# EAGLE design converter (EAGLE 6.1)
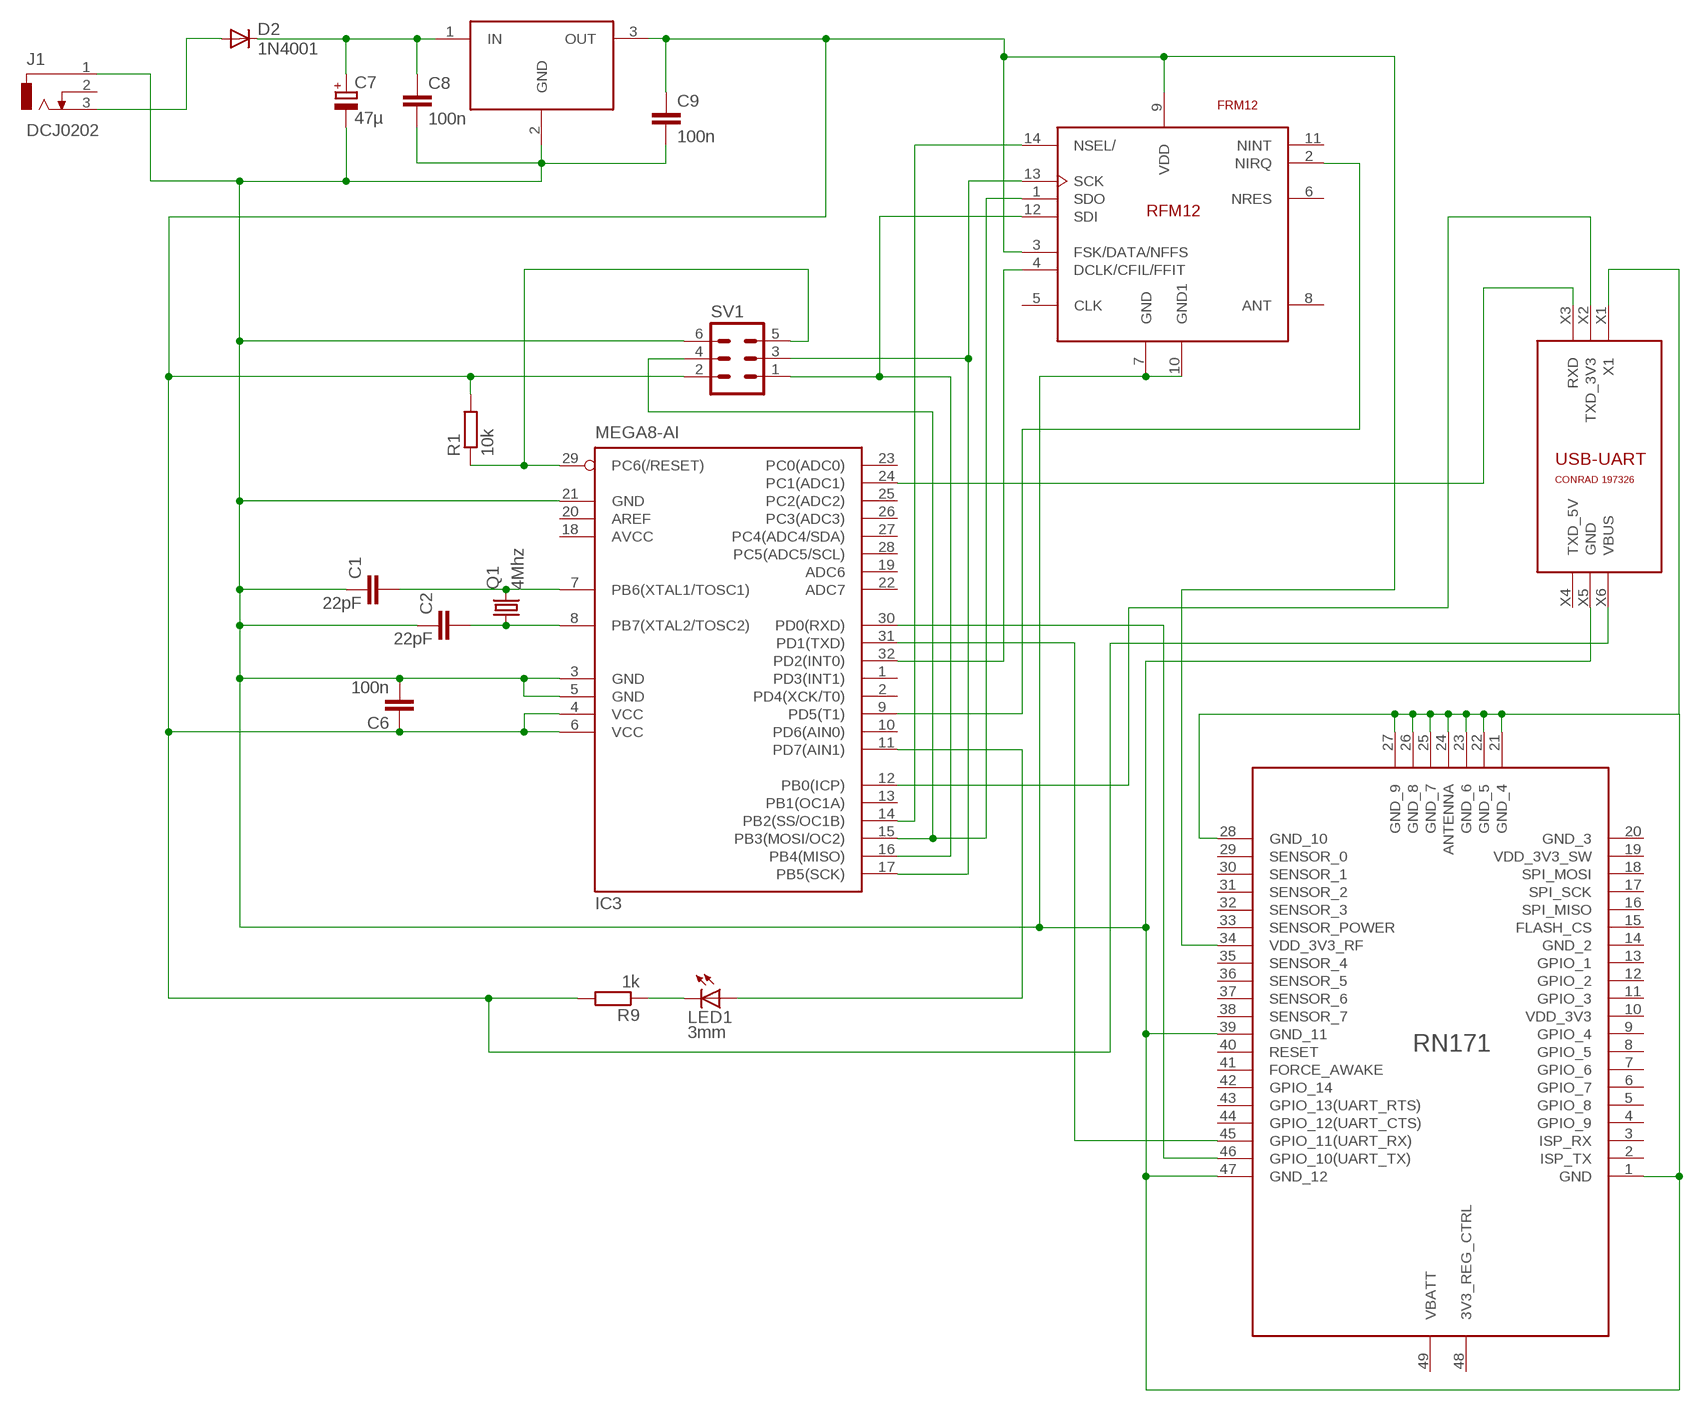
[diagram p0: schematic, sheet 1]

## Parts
C1  22pF  C-EUC0603  [C0603]
C2  22pF  C-EUC0603  [C0603]
C6  100n  C-EUC0603  [C0603]
C7  47µ  CPOL-EUC  [PANASONIC_C]
C8  100n  C-EUC0603  [C0603]
C9  100n  C-EUC0603  [C0603]
D2  1N4001  CGRM4001-G  [SOD-123_MINI-SMA]
IC3  MEGA8-AI  [TQFP32-08]
J1  DCJ0202  [DCJ0202]
LED1  3mm  LED3MM  [LED3MM]
Q1  4Mhz  CRYSTALHC49UP  [HC49UP]
R1  10k  R-EU_R0603  [R0603]
R9  1k  R-EU_R0603  [R0603]
SV1  ML6  [ML6]
U$1  FRM12  [RFM12]
U$2  LM3940IMP-3.3  [SOT223]
U$3  USB-UART  [USB-UART]
U$4  RN171  [RN171]

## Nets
GND: C1.1 C2.1 C6.2 C7.- C8.2 C9.2 IC3.3(GND) IC3.5(GND) IC3.21(GND) J1.1 SV1.6 U$1.7(GND) U$1.10(GND1) U$2.2(GND) U$3.X1 U$3.X5(GND) U$4.1(GND) U$4.21(GND_4) U$4.22(GND_5) U$4.23(GND_6) U$4.24(ANTENNA) U$4.25(GND_7) U$4.26(GND_8) U$4.27(GND_9) U$4.28(GND_10) U$4.39(GND_11) U$4.47(GND_12)
IN: C7.+ C8.1 D2.C U$2.1(IN)
N$1: C1.2 IC3.7(PB6(XTAL1/TOSC1)) Q1.2
N$2: C2.2 IC3.8(PB7(XTAL2/TOSC2)) Q1.1
N$4: D2.A J1.3
N$5: IC3.29(PC6(/RESET)) R1.1 SV1.5
N$7: IC3.15(PB3(MOSI/OC2)) SV1.4 U$1.1(SDO)
N$8: IC3.16(PB4(MISO)) SV1.1 U$1.12(SDI)
N$11: IC3.32(PD2(INT0)) U$1.4(DCLK/CFIL/FFIT)
N$12: IC3.14(PB2(SS/OC1B)) U$1.14(NSEL/)
N$13: IC3.9(PD5(T1)) U$1.2(NIRQ)
N$14: IC3.11(PD7(AIN1)) LED1.A
N$15: LED1.K(C) R9.1
N$16: IC3.17(PB5(SCK)) SV1.3 U$1.13(SCK)
N$18: IC3.31(PD1(TXD)) U$4.45(GPIO_11(UART_RX))
N$19: IC3.30(PD0(RXD)) U$4.46(GPIO_10(UART_TX))
N$20: IC3.12(PB0(ICP)) U$3.X2(TXD_3V3)
N$22: IC3.24(PC1(ADC1)) U$3.X3(RXD)
VCC: C6.1 C9.1 IC3.4(VCC) IC3.6(VCC) R1.2 R9.2 SV1.2 U$1.3(FSK/DATA/NFFS) U$1.9(VDD) U$2.3(OUT) U$3.X6(VBUS) U$4.34(VDD_3V3_RF)
Unconnected: IC3.1(PD3(INT1)) IC3.2(PD4(XCK/T0)) IC3.10(PD6(AIN0)) IC3.13(PB1(OC1A)) IC3.19(ADC6) IC3.20(AREF) IC3.22(ADC7) IC3.23(PC0(ADC0)) IC3.25(PC2(ADC2)) IC3.26(PC3(ADC3)) IC3.27(PC4(ADC4/SDA)) IC3.28(PC5(ADC5/SCL)) J1.2 U$1.5(CLK) U$1.6(NRES) U$1.8(ANT) U$1.11(NINT) U$3.X4(TXD_5V) U$4.2(ISP_TX) U$4.3(ISP_RX) U$4.4(GPIO_9) U$4.5(GPIO_8) U$4.6(GPIO_7) U$4.7(GPIO_6) U$4.8(GPIO_5) U$4.9(GPIO_4) U$4.10(VDD_3V3) U$4.11(GPIO_3) U$4.12(GPIO_2) U$4.13(GPIO_1) U$4.14(GND_2) U$4.15(FLASH_CS) U$4.16(SPI_MISO) U$4.17(SPI_SCK) U$4.18(SPI_MOSI) U$4.19(VDD_3V3_SW) U$4.20(GND_3) U$4.29(SENSOR_0) U$4.30(SENSOR_1) U$4.31(SENSOR_2) U$4.32(SENSOR_3) U$4.33(SENSOR_POWER) U$4.35(SENSOR_4) U$4.36(SENSOR_5) U$4.37(SENSOR_6) U$4.38(SENSOR_7) U$4.40(RESET) U$4.41(FORCE_AWAKE) U$4.42(GPIO_14) U$4.43(GPIO_13(UART_RTS)) U$4.44(GPIO_12(UART_CTS)) U$4.48(3V3_REG_CTRL) U$4.49(VBATT)

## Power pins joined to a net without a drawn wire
AVCC: IC3.18(AVCC)

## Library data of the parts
C1 C2 C6 C8 C9 = rcl:C-EU: CAPACITOR, European symbol
C7 = rcl:CPOL-EU: POLARIZED CAPACITOR, European symbol
D2 = diode:CGRM400*-G: Molded plasitc,JEDEC SOD-123/Mini SMA
IC3 = atmel:MEGA8: MICROCONTROLLER 8 Kbytes FLASH, 1 kbytes SRAM, 512 bytes EEPROM, USART, 6-channel 10 bit ADC, 2-channel 8 bit ADC Pin compatible with Atmega48, ATMega88, ATMega168 Source: avr.lbr; MPN: ATMEGA8-16AU; OC_FARNELL: 9171371; OC_NEWARK: 73M8863
J1 = con-jack:DCJ0202: DC POWER JACK Source: DCJ0202.pdf; OC_FARNELL: unknown; OC_NEWARK: unknown
LED1 = led:LED: LED
Q1 = crystal:CRYSTAL: CRYSTAL; OC_FARNELL: unknown; OC_NEWARK: unknown
R1 R9 = rcl:R-EU_: RESISTOR, European symbol
SV1 = con-ml:ML6: HARTING; OC_FARNELL: unknown; OC_NEWARK: unknown
U$1 = RFM12:FRM12
U$2 = LM3940:LM3940IMP-3.3: 1A Low Dropout Regulator for 5V to 3.3V Conversion
U$3 = usb-uart:USB-UART
U$4 = RN171:RN171: RN171

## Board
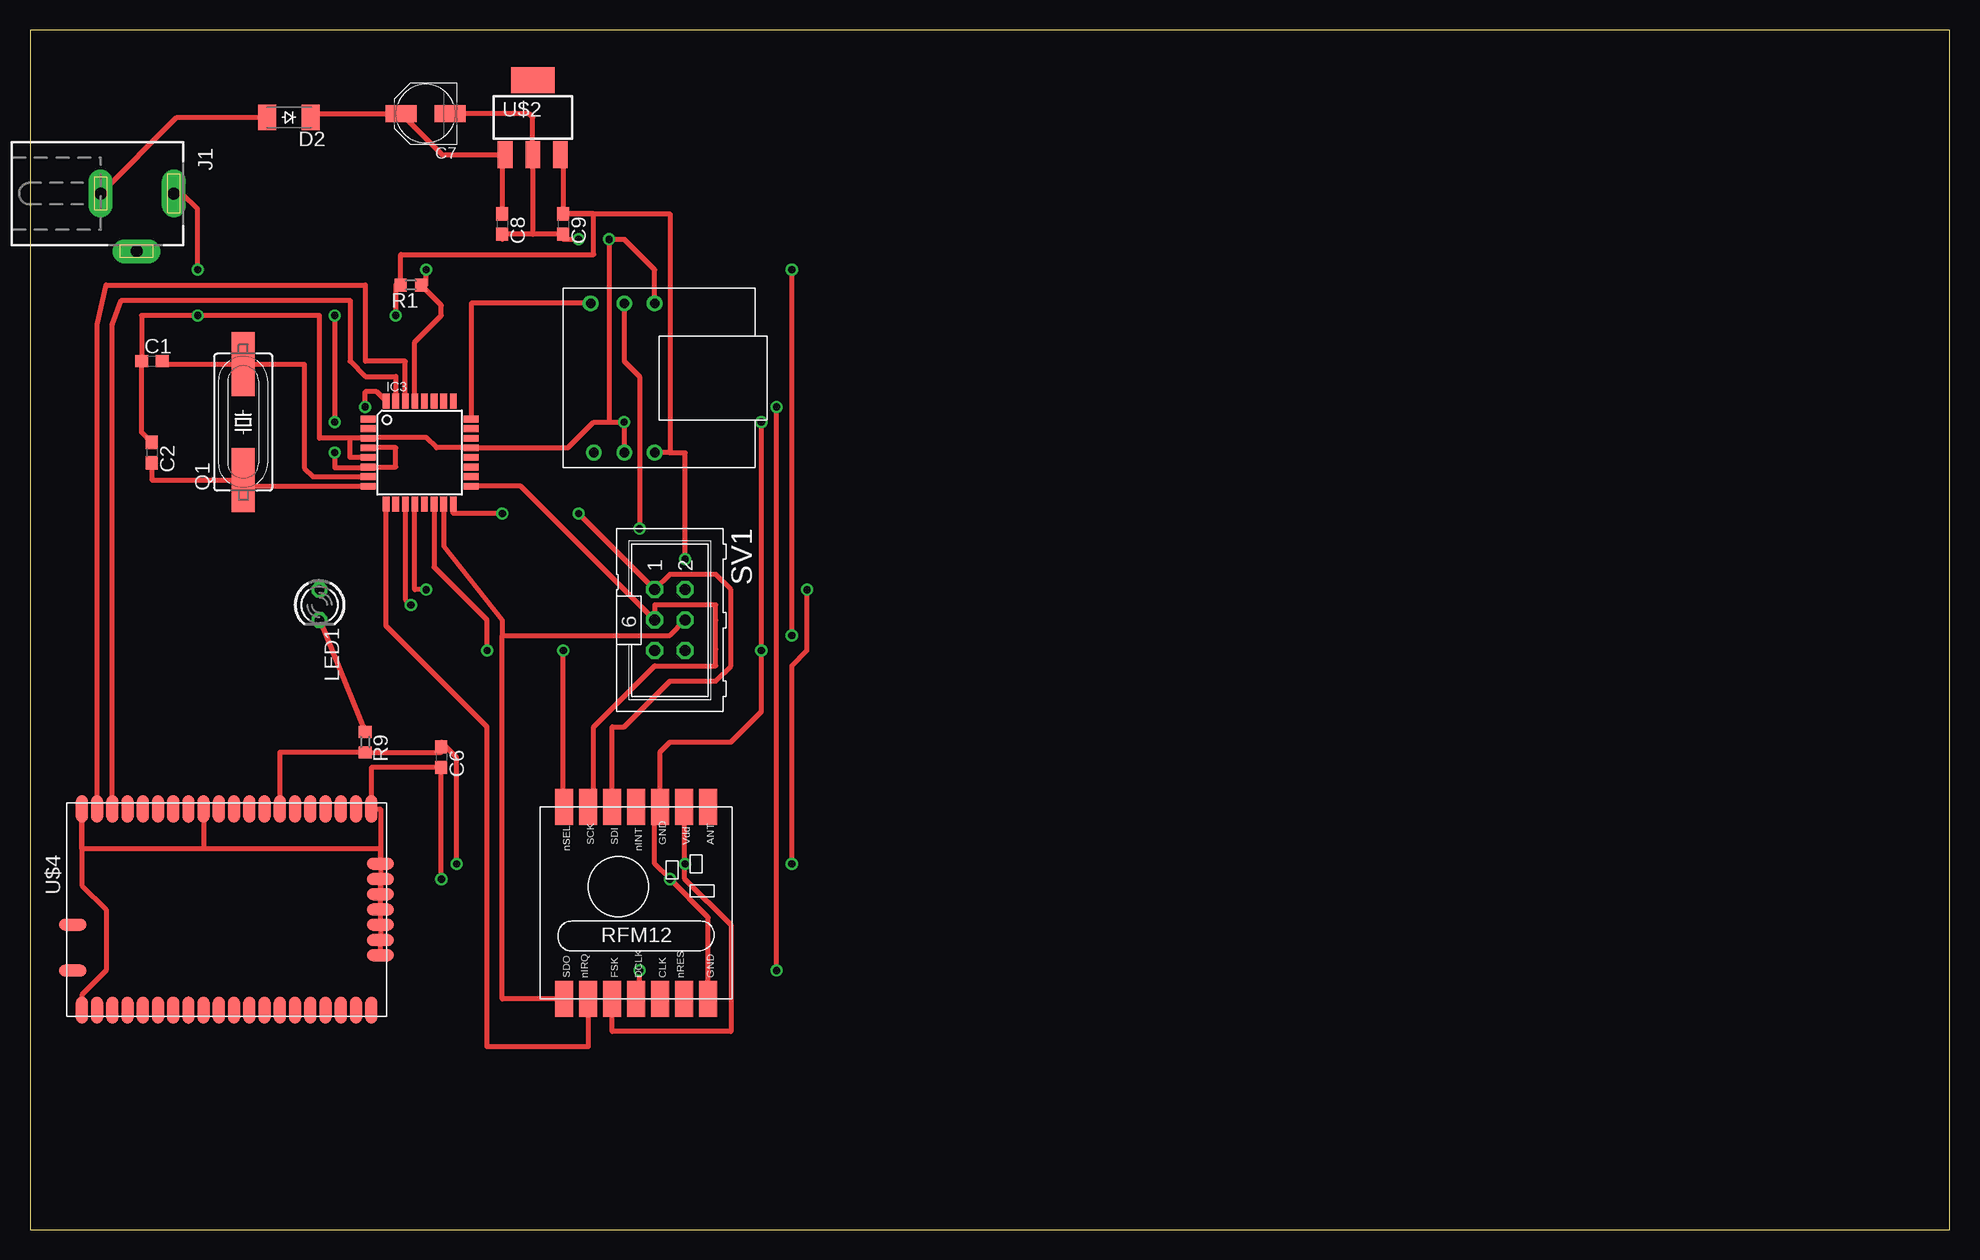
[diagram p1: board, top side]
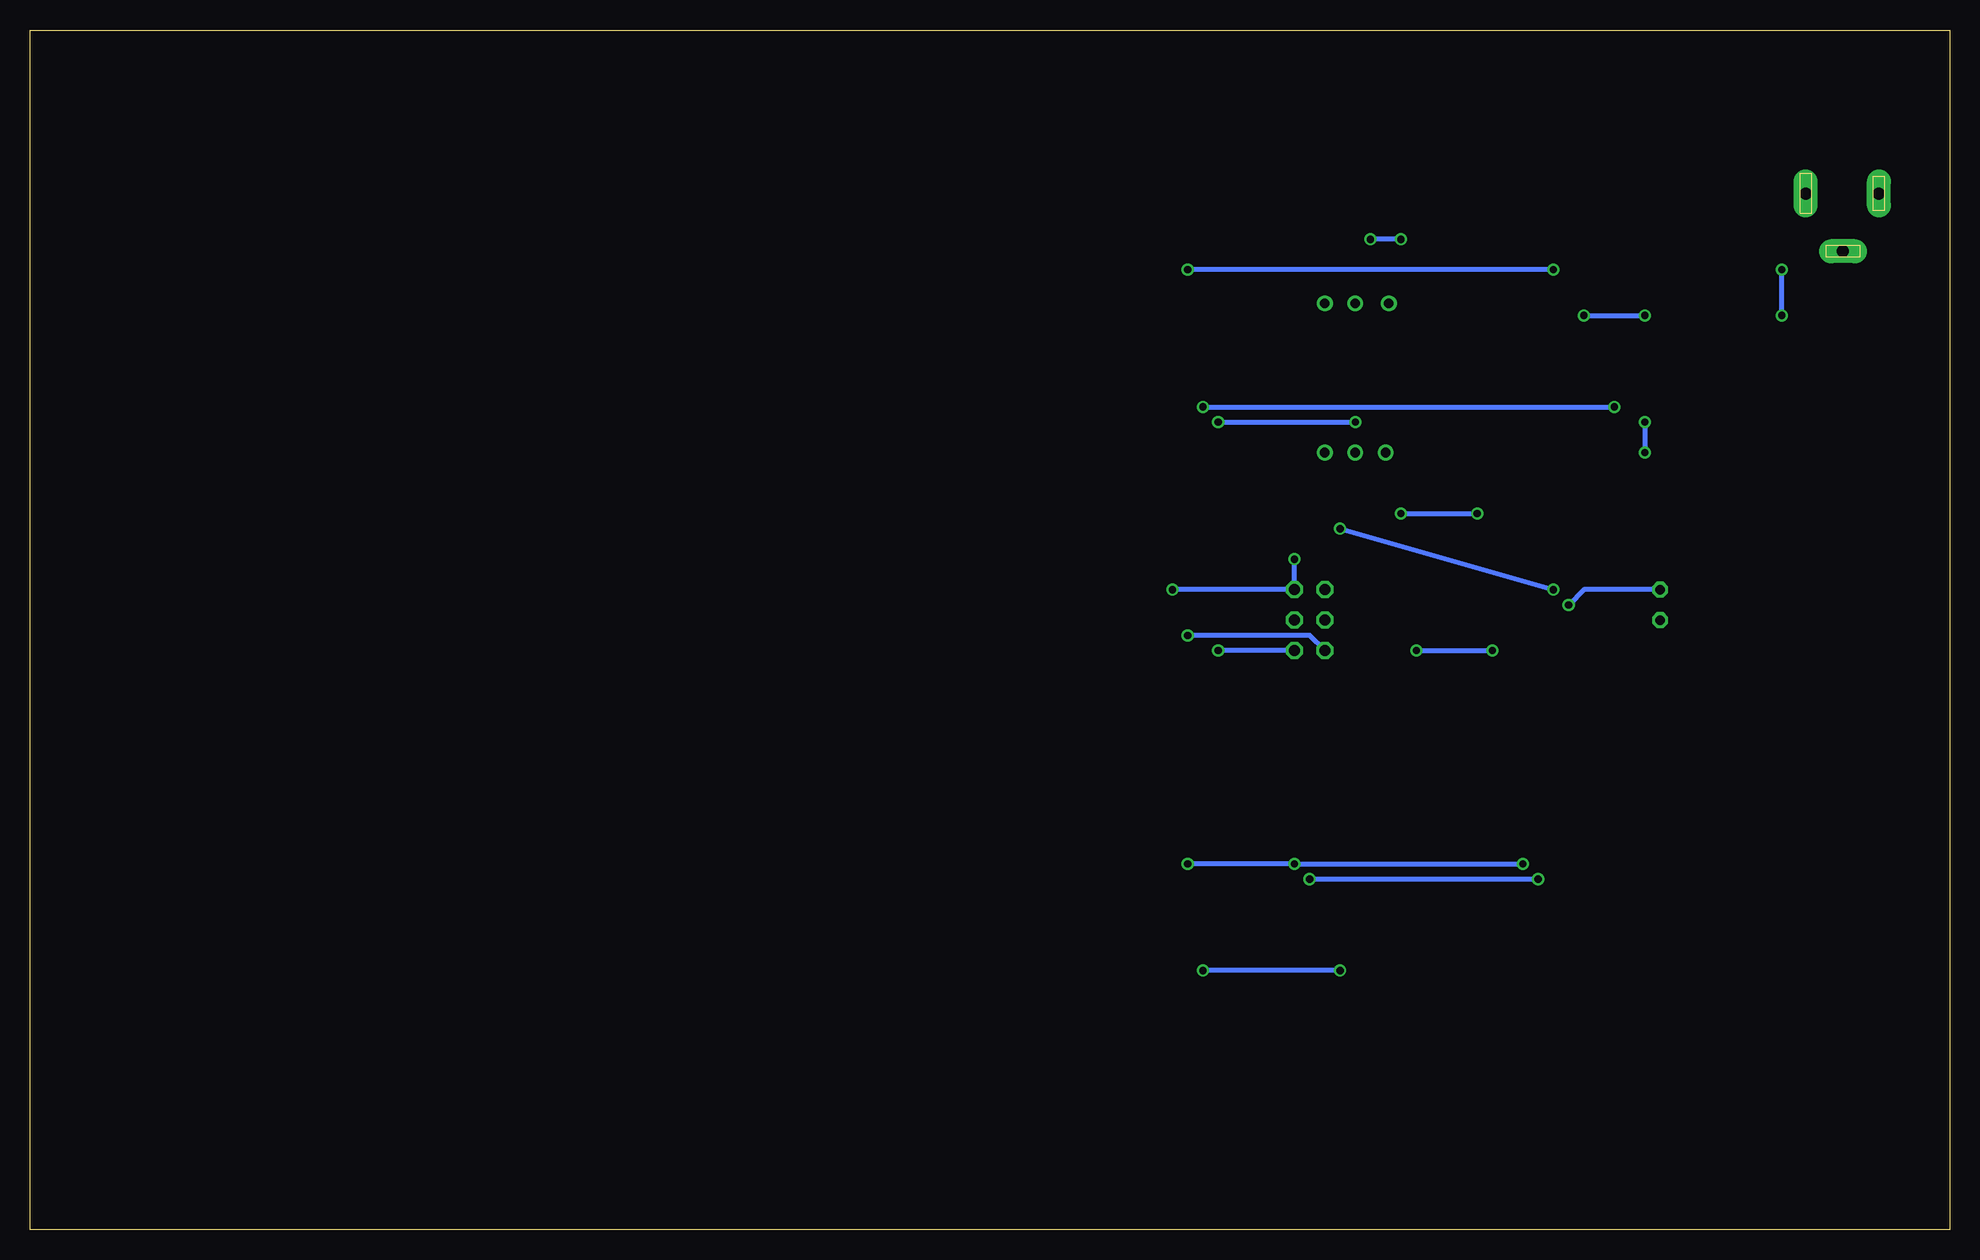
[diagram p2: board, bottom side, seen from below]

Size 160 x 100 mm. Coordinates in mm from the lower left corner, seen from the top.
Outline: 0,0 160,0 160,100 0,100 0,0
Copper layers (1*16): Top 0.035mm / dielectric 1.5mm / Bottom 0.035mm
Design rules: minimum track width 10mil, minimum drill 20mil, track to track 8mil, track to pad 8mil, pad to pad 8mil, via to via 8mil, smd to smd 8mil, copper to edge 40mil, drill to drill 8mil, minimum pad ring 10mil, minimum via ring 8mil, stop-mask expansion 4mil, vias tented up to drill 0mil, thermal gap 10mil

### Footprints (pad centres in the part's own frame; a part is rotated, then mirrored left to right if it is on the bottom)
C0603 = smd 1.1 x 1: 1 -0.85,0; 2 0.85,0
PANASONIC_C = smd 2.6 x 1.4: + 2.05,0; - -2.05,0
SOD-123_MINI-SMA = smd 1.5 x 2.1: A 1.8,0; C -1.8,0
TQFP32-08 = smd 1.27 x 0.559: 1 -4.293,2.8; 2 -4.293,2; 3 -4.293,1.2; 4 -4.293,0.4; 5 -4.293,-0.4; 6 -4.293,-1.2; 7 -4.293,-2; 8 -4.293,-2.8; 17 4.293,-2.8; 18 4.293,-2; 19 4.293,-1.2; 20 4.293,-0.4; 21 4.293,0.4; 22 4.293,1.2; 23 4.293,2; 24 4.293,2.8 | smd 0.559 x 1.27: 9 -2.8,-4.293; 10 -2,-4.293; 11 -1.2,-4.293; 12 -0.4,-4.293; 13 0.4,-4.293; 14 1.2,-4.293; 15 2,-4.293; 16 2.8,-4.293; 25 2.8,4.293; 26 2,4.293; 27 1.2,4.293; 28 0.4,4.293; 29 -0.4,4.293; 30 -1.2,4.293; 31 -2,4.293; 32 -2.8,4.293
DCJ0202 = drill 1 pad 2 long: 1 0,3.1; 2 4.8,0; 3 0,-3
LED3MM = drill 0.813 octagon: A -1.27,0; K 1.27,0
HC49UP = smd 5.334 x 1.93: 1 -4.826,0; 2 4.826,0
R0603 = smd 1 x 1.1: 1 -0.85,0; 2 0.85,0
ML6 = drill 0.914 octagon: 1 -2.54,-1.27; 2 -2.54,1.27; 3 0,-1.27; 4 0,1.27; 5 2.54,-1.27; 6 2.54,1.27
RFM12 = smd 1.5 x 3: 1 -5,-10; 2 -3,-10; 3 -1,-10; 4 1,-10; 5 3,-10; 6 5,-10; 7 7,-10; 8 7,6; 9 5,6; 10 3,6; 11 1,6; 12 -1,6; 13 -3,6; 14 -5,6
SOT223 = smd 1.219 x 2.235: 1 -2.311,-3.099; 2 0,-3.099; 3 2.311,-3.099 | smd 3.6 x 2.2: 4 0,3.099
USB-UART = drill 0.8: X1 1.27,6.096; X2 -1.27,6.096; X3 -4.064,6.096; X4 -3.81,-6.35; X5 -1.27,-6.35; X6 1.27,-6.35
RN171 = smd 1.016 x 2.286: 1 12.192,8.382; 2 10.922,8.382; 3 9.652,8.382; 4 8.382,8.382; 5 7.112,8.382; 6 5.842,8.382; 7 4.572,8.382; 8 3.302,8.382; 9 2.032,8.382; 10 0.762,8.382; 11 -0.508,8.382; 12 -1.778,8.382; 13 -3.048,8.382; 14 -4.318,8.382; 15 -5.588,8.382; 16 -6.858,8.382; 17 -8.128,8.382; 18 -9.398,8.382; 19 -10.668,8.382; 20 -11.938,8.382; 28 -11.938,-8.382; 29 -10.668,-8.382; 30 -9.398,-8.382; 31 -8.128,-8.382; 32 -6.858,-8.382; 33 -5.588,-8.382; 34 -4.318,-8.382; 35 -3.048,-8.382; 36 -1.778,-8.382; 37 -0.508,-8.382; 38 0.762,-8.382; 39 2.032,-8.382; 40 3.302,-8.382; 41 4.572,-8.382; 42 5.842,-8.382; 43 7.112,-8.382; 44 8.382,-8.382; 45 9.652,-8.382; 46 10.922,-8.382; 47 12.192,-8.382 | smd 2.286 x 1.016: 21 -12.7,3.81; 22 -12.7,2.54; 23 -12.7,1.27; 24 -12.7,0; 25 -12.7,-1.27; 26 -12.7,-2.54; 27 -12.7,-3.81; 48 12.954,5.08; 49 12.954,1.27

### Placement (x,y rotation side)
C1  10.16,72.39 0 top
C2  10.16,64.77 270 top
C6  34.29,39.37 270 top
C7  32.98,93.02 180 top
C8  39.37,83.82 270 top
C9  44.45,83.82 270 top
D2  21.59,92.71 180 top
IC3  32.48,64.77 0 top
J1  8.89,86.36 270 top
LED1  24.13,52.07 270 top
Q1  17.78,67.31 90 top
R1  31.75,78.74 180 top
R9  27.94,40.64 270 top
SV1  53.34,50.8 270 top
U$1  49.53,29.21 0 top
U$2  41.91,92.71 0 top
U$3  50.8,71.12 0 top
U$4  16.51,26.67 180 top

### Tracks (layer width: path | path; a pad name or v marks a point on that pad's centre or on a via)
GND  (via drill 0.6)
  Top 0.406: C2.1 9.31,66.47 C1.1 9.31,76.2 v13.97,76.2 24.13,76.2 24.13,65.97 26.67,65.97 | 26.67,65.97 IC3.3 28.26,66.04 33.02,66.04 33.89,65.17 IC3.21 44.85,65.17 46.99,67.31 48.26,67.31 | C7.- 41.6,93.02 41.91,92.71 U$2.2 41.91,82.97 | 41.91,82.97 C9.2 44.45,82.55 v45.72,82.55 | 41.91,82.97 C8.2 39.37,82.55 | U$4.21 U$4.22 U$4.23 U$4.24 U$4.25 | U$4.25 U$4.26 | U$4.27 U$4.25 | U$4.27 29.21,31.75 14.48,31.75 | U$4.27 29.21,35.05 U$4.28 28.45,38.52 C6.2 v34.29,29.21 | U$4.39 14.48,31.75 | 14.48,31.75 4.32,31.75 U$4.47 4.32,28.7 6.35,26.67 6.35,21.59 4.32,19.56 U$4.1 | IC3.5 26.67,64.37 26.67,65.97 | U$3.X5 v49.53,67.31 48.26,67.31 | v60.96,67.31 v60.96,48.26 60.96,43.18 58.42,40.64 53.34,40.64 52.53,39.83 U$1.10 52.07,34.75 52.07,30.48 v53.34,29.21 56.53,26.02 U$1.7 | 48.26,67.31 v48.26,82.55 49.53,82.55 52.07,80.01 U$3.X1 | J1.1 12.7,86.36 13.97,85.09 v13.97,80.01
  Bottom 0.406: v60.96,67.31 v49.53,67.31 | SV1.6 v60.96,48.26 | v53.34,29.21 v34.29,29.21 | v45.72,82.55 v48.26,82.55 | v13.97,76.2 v13.97,80.01
IN
  Top 0.406: D2.C 23.7,93.02 C7.+ 34.34,89.61 U$2.1 39.37,89.38 C8.1
N$1
  Top 0.406: C1.2 11.01,72.14 Q1.2 22.86,72.14 22.86,63.5 23.59,62.77 IC3.7
N$2
  Top 0.406: C2.2 10.16,62.48 Q1.1 17.78,61.97 IC3.8
N$4
  Top 0.406: J1.3 12.24,92.71 D2.A
N$5  (via drill 0.6)
  Top 0.406: IC3.29 32.08,73.99 34.29,76.2 34.29,77.05 R1.1 33.02,78.74 v33.02,80.01 | v63.5,49.53 v63.5,80.01
  Bottom 0.406: v33.02,80.01 v63.5,80.01 | v63.5,49.53 53.34,49.53 SV1.5
N$7
  Top 0.406: U$1.1 39.37,19.21 39.37,49.53 | IC3.15 34.48,56.96 39.37,50.8 39.37,49.53 | 39.37,49.53 53.34,49.53 SV1.4
N$8  (via drill 0.6)
  Top 0.406: U$1.12 48.53,41.91 49.53,41.91 53.34,45.72 57.15,45.72 58.42,46.99 58.42,53.34 57.15,54.61 53.34,54.61 SV1.1 v45.72,59.69 | v39.37,59.69 35.28,59.69 IC3.16
  Bottom 0.406: v45.72,59.69 v39.37,59.69
N$11  (via drill 0.6)
  Top 0.406: v62.23,21.59 v62.23,68.58 | v50.8,21.59 50.8,20.32 U$1.4 | v27.94,68.58 27.94,69.85 28.89,69.85 IC3.32
  Bottom 0.406: v62.23,68.58 v27.94,68.58 | v50.8,21.59 v62.23,21.59
N$12  (via drill 0.6)
  Top 0.406: v38.1,48.26 38.1,50.8 33.68,55.22 IC3.14 | v44.45,48.26 44.45,35.56 U$1.14
  Bottom 0.406: v44.45,48.26 v38.1,48.26
N$13
  Top 0.406: U$1.2 46.53,15.24 38.1,15.24 38.1,41.91 29.68,50.33 IC3.9
N$14  (via drill 0.6)
  Top 0.406: IC3.11 31.28,52.54 v31.75,52.07
  Bottom 0.406: v31.75,52.07 30.48,53.34 LED1.A
N$15
  Top 0.406: LED1.K R9.1
N$16
  Top 0.406: IC3.17 40.9,61.97 SV1.3 52.07,52.07 57.15,52.07 57.15,50.8 57.15,48.37 57.15,46.99 52.07,46.99 46.99,41.91 46.99,35.67 U$1.13
N$18
  Top 0.406: U$4.45 6.86,75.44 7.62,77.47 26.67,77.47 26.67,72.39 27.94,71.12 30.48,71.12 IC3.31
N$19
  Top 0.406: U$4.46 5.59,75.44 6.35,78.74 27.94,78.74 27.94,72.39 31.28,72.39 IC3.30
N$20  (via drill 0.6)
  Top 0.406: v33.02,53.34 32.08,53.34 IC3.12 | v50.8,58.42 50.8,71.12 49.53,72.39 U$3.X2 49.53,77.47
  Bottom 0.406: v50.8,58.42 v33.02,53.34
N$22
  Top 0.406: U$3.X3 36.77,77.22 IC3.24
VCC  (via drill 0.6)
  Top 0.406: IC3.6 27.94,63.57 27.94,63.5 | U$2.3 44.45,89.38 C9.1 | v25.4,64.77 25.4,63.5 27.94,63.5 | v25.4,76.2 v25.4,67.31 | v30.48,76.2 30.48,78.74 R1.2 30.9,81.28 46.99,81.28 46.99,84.67 C9.1 | 27.94,63.5 IC3.6 | IC3.6 30.48,63.57 30.48,65.17 IC3.4 | U$1.9 54.53,30.48 | 54.53,30.48 54.53,29.29 58.42,25.4 58.42,16.51 48.53,16.51 U$1.3 | U$4.34 20.83,39.79 R9.2 34.29,39.79 C6.1 34.29,40.64 35.56,39.37 v35.56,30.48 | v54.61,30.48 54.53,30.48 | C9.1 53.34,84.67 53.34,64.77 | 53.34,64.77 U$3.X6 | v54.61,55.88 54.61,64.77 53.34,64.77 | v64.77,53.34 64.77,48.26 63.5,46.99 v63.5,30.48
  Bottom 0.406: v25.4,67.31 v25.4,64.77 | v30.48,76.2 v25.4,76.2 | v35.56,30.48 v54.61,30.48 v63.5,30.48 | v54.61,55.88 SV1.2 v64.77,53.34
